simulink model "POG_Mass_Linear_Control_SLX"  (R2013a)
settings: Solver=ode45  StartTime=0.0  StopTime=10.0  MaxStep=0.001  RelTol=1e-3
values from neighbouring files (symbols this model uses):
  Kp = 10000    [POG_Mass_Linear_Control_SLX_m.m]
  Nc = 30*Newton    (= 30)    [POG_Mass_Linear_Control_SLX_m.m]    (also in POG_Mechanical_system_J_K_T_M_K_NL_SLX_m.m = 2)
  tau1 = (M0-cos(Ph0))/(w*sin(Ph0))    [POG_Mass_Linear_Control_SLX_m.m]
  tau2 = (cos(Ph0)-1/M0)/(w*sin(Ph0))    [POG_Mass_Linear_Control_SLX_m.m]
  Ts = Tfin/Nr_Ts_Points    (= 0.0025)    [POG_Mechanical_system_J_K_T_M_K_Par_SLX_m.m]    (also in POG_Mechanical_system_J_K_T_M_K_SLX_m.m = 0.005; POG_Mechanical_system_J_K_T_M_K_SuperBlock_SLX_m.m = 0.005; POG_Mass_Linear_Control_SLX_m.m; POG_Mechanical_system_J_K_T_M_K_NL_SLX_m.m)
  Vx0 = 0    [POG_Mechanical_system_J_K_T_M_K_NL_SLX_m.m]
  x_0 = 0    [POG_Mass_Linear_Control_SLX_m.m]
  x_r = 1*meters    (= 1)    [POG_Mass_Linear_Control_SLX_m.m]
undefined symbols (not defined in the file or in its folder): b, m

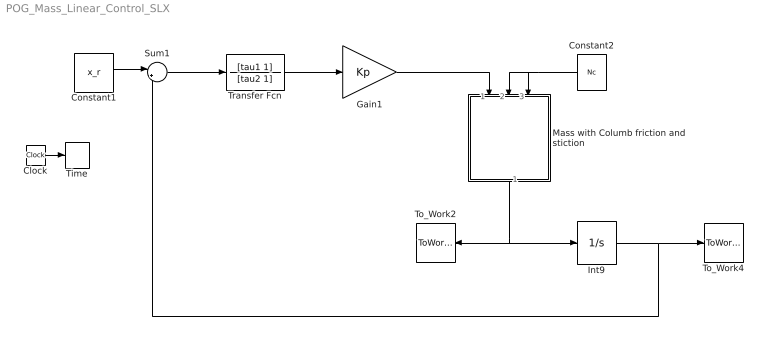
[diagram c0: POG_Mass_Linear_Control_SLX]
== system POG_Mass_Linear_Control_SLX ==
  Clock : Clock
  Constant1 : Constant  Value=x_r
  Constant2 : Constant  Value=Nc
  Gain1 : Gain  Gain=Kp
  Int9 : Integrator  InitialCondition=x_0
  Mass with Columb friction and stiction : Subsystem
  Sum1 : Sum  Inputs=|+-
  Time : ToWorkspace  VariableName=t  SampleTime=Ts
  To_Work2 : ToWorkspace  VariableName=w_m  SampleTime=Ts
  To_Work4 : ToWorkspace  VariableName=x  SampleTime=Ts
  Transfer Fcn : TransferFcn  Numerator=[tau1 1]  Denominator=[tau2 1]
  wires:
  Clock/1 -> Time/1
  Constant1/1 -> Sum1/1
  Sum1/1 -> Transfer Fcn/1
  Gain1/1 -> Mass with Columb friction and stiction/1(F)
  Int9/1 -> Sum1/2, To_Work4/1
  Transfer Fcn/1 -> Gain1/1
  Mass with Columb friction and stiction/1(Vx) -> Int9/1, To_Work2/1
  Constant2/1 -> Mass with Columb friction and stiction/3(Ns), Mass with Columb friction and stiction/2(Nc)

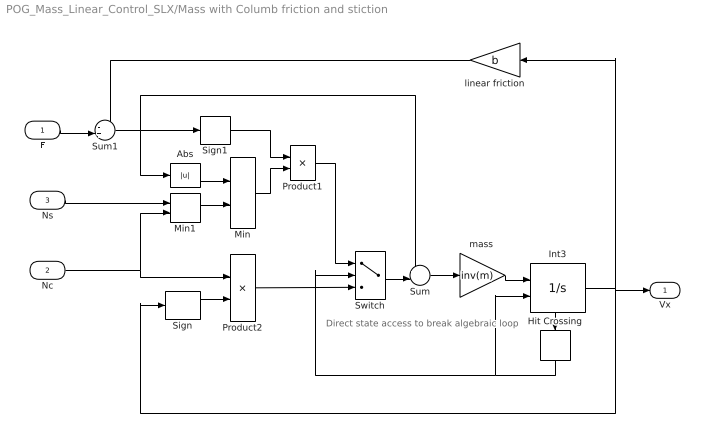
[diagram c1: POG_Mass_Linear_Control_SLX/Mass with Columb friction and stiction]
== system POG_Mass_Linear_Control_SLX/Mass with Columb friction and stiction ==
  note: Direct state access to break algebraic loop
  F : Inport
  Nc : Inport  Port=2
  Ns : Inport  Port=3
  Abs : Abs
  Hit Crossing : HitCross
  Int3 : Integrator  ExternalReset=rising  InitialCondition=Vx0  ShowStatePort=on
  Min : MinMax  Inputs=2
  Min1 : MinMax  Function=max  Inputs=2
  Product1 : Product
  Product2 : Product
  Sign : Signum
  Sign1 : Signum
  Sum : Sum  Inputs=+-|
  Sum1 : Sum  Inputs=-+|
  Switch : Switch  Threshold=0.5
  linear friction : Gain  Gain=b
  "mass " : Gain  Gain=inv(m)
  Vx : Outport  InitialOutput=0
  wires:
  F/1 -> Sum1/2
  linear friction/1 -> Sum1/1
  Ns/1 -> Min1/1
  Min1/1 -> Min/2
  Abs/1 -> Min/1
  Min/1 -> Product1/2
  Sign1/1 -> Product1/1
  Sign/1 -> Product2/2
  Nc/1 -> Min1/2, Product2/1
  Product2/1 -> Switch/3
  Int3/1 -> linear friction/1, Sign/1, Vx/1
  Int3/State -> Hit Crossing/1
  "mass "/1 -> Int3/1
  Sum/1 -> "mass "/1
  Sum1/1 -> Sign1/1, Abs/1, Sum/1
  Hit Crossing/1 -> Int3/2, Switch/2
  Switch/1 -> Sum/2
  Product1/1 -> Switch/1
